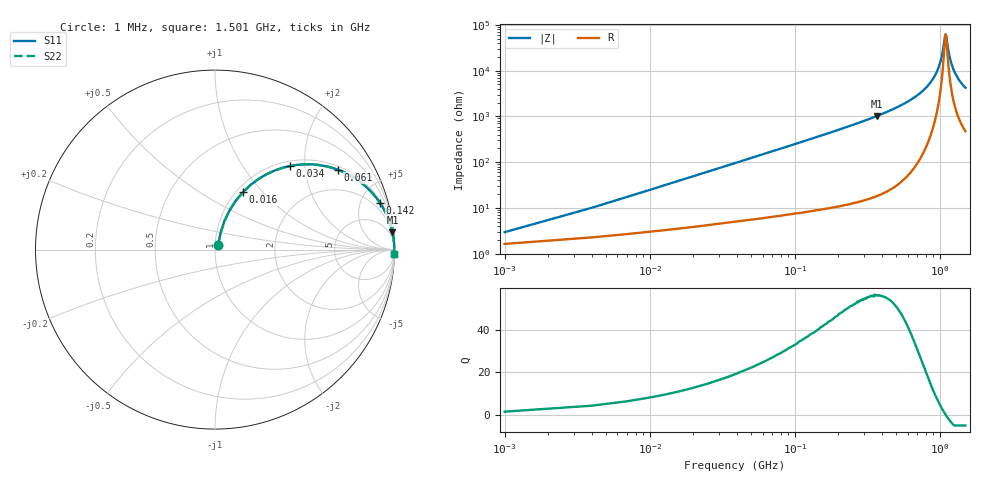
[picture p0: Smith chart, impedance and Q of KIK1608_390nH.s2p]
!version-2
!date-01.2022
!Series
# MHz S RI R 50
!Freq ReS11 ImS11 ReS21 ImS21 ReS12 ImS12 ReS22 ImS22
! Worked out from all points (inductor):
!   501 points, 1 MHz to 1.501 GHz, reference 50 ohm
!   read as one part in series: L = 390 nH near 7 MHz
!   highest Q = 56.4 at 367 MHz (marker M1), where L = 439 nH
!   self-resonance near 1.096 GHz
!   S11 on the Smith chart (normalised r, x): 1 MHz: 1.03, +0.05; 16 MHz: 1.07, +0.78; 34 MHz: 1.09, +1.67; 61 MHz: 1.12, +3.00; 142 MHz: 1.18, +7.08; 1.501 GHz: 10, -84
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1  0.0166 0.0237  0.9834 -0.0237  0.9834 -0.0237  0.0166 0.0237
10  0.0812 0.2186  0.9188 -0.2186  0.9188 -0.2186  0.0812 0.2186
16  0.1553 0.3199  0.8447 -0.3199  0.8447 -0.3199  0.1553 0.3199
25  0.2869 0.4195  0.7131 -0.4195  0.7131 -0.4195  0.2869 0.4195
34  0.4156 0.4654  0.5844 -0.4654  0.5844 -0.4654  0.4156 0.4654
61  0.6856 0.4447  0.3144 -0.4447  0.3144 -0.4447  0.6856 0.4447
94  0.8359 0.3551  0.1641 -0.3551  0.1641 -0.3551  0.8359 0.3551
142  0.9206 0.2581  0.0794 -0.2581  0.0794 -0.2581  0.9206 0.2581
253  0.9745 0.1483  0.0255 -0.1483  0.0255 -0.1483  0.9745 0.1483
367  0.9886 0.0974  0.0114 -0.0974  0.0114 -0.0974  0.9886 0.0974
502  0.9946 0.0638  0.00536 -0.0638  0.00536 -0.0638  0.9946 0.0638
751  0.998 0.0288  0.00198 -0.0288  0.00198 -0.0288  0.998 0.0288
904  0.9985 0.0145  0.0015 -0.0145  0.0015 -0.0145  0.9985 0.0145
1003  0.9985 0.0067  0.00148 -0.0067  0.00148 -0.0067  0.9985 0.0067
1042  0.9985 0.00387  0.00152 -0.00387  0.00152 -0.00387  0.9985 0.00387
1087  0.9984 0.000734  0.0016 -0.000734  0.0016 -0.000734  0.9984 0.000734
1099  0.9984 -7.86e-05  0.00162 7.86e-05  0.00162 7.86e-05  0.9984 -7.86e-05
1171  0.9982 -0.00477  0.00179 0.00477  0.00179 0.00477  0.9982 -0.00477
1207  0.9981 -0.00702  0.0019 0.00702  0.0019 0.00702  0.9981 -0.00702
1252  0.9979 -0.00974  0.00206 0.00974  0.00206 0.00974  0.9979 -0.00974
1357  0.9975 -0.0158  0.00249 0.0158  0.00249 0.0158  0.9975 -0.0158
1501  0.9968 -0.0234  0.00321 0.0234  0.00321 0.0234  0.9968 -0.0234
